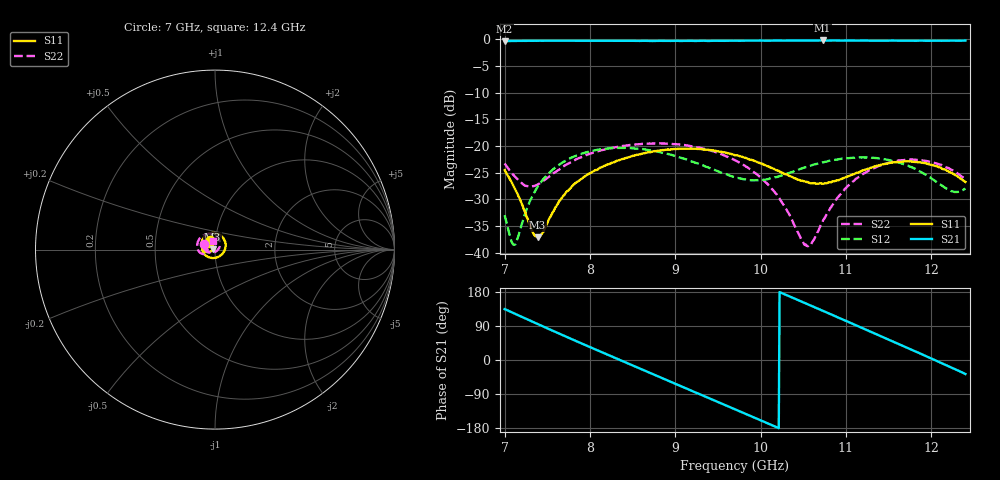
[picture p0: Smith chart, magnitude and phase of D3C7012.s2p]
! 11/4/2020 3:57:07 PM
! C:\USERS\DITOM\DESKTOP\SINGLE JUNCTION ISOLATOR DATA\7.0 - 12.4 GHZ (D3I7012).S2P
! CHANNEL.1
! TR.MEASUREMENT
! CORRECTED.DATA
# GHZ S RI R 50.0
! FREQ.GHZ  S11RE  S11IM  S21RE  S21IM  S12RE  S12IM  S22RE  S22IM
!; PortSelection: Port_12
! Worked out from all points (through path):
!   601 points, 7 GHz to 12.4 GHz, reference 50 ohm
!   highest |S21| = -0.23 dB at 10.73 GHz (marker M1); lowest = -0.4 dB at 7 GHz (marker M2)
!   lowest |S11| = -37.1 dB at 7.387 GHz (marker M3), VSWR 1.03, Z = 48.7 + j0.403 ohm
!   |S11| at or under -10 dB: start of sweep to end of sweep
!   |S22| runs from -38.8 to -19.5 dB; largest |S21 - S12| = 0.98
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7  -0.0303 0.0511  -0.6701 0.6869  0.0224 0.00224  -0.0619 0.0295
7.126  -0.0173 0.0352  -0.5027 0.8218  0.00612 0.0103  -0.0483 0.0174
7.387  -0.0133 0.00413  -0.0823 0.964  0.00224 0.0414  -0.0423 -0.00948
7.639  -0.0279 -0.0123  0.3367 0.908  0.0316 0.0588  -0.0554 -0.0235
7.9  -0.0474 -0.0131  0.6976 0.6714  0.0718 0.0449  -0.0754 -0.022
8.134  -0.063 -0.00263  0.9034 0.3469  0.093 0.00845  -0.0909 -0.00903
8.341  -0.0724 0.0134  0.9661 0.0136  0.0908 -0.0306  -0.0982 0.00975
8.593  -0.0744 0.0389  0.8853 -0.3841  0.0647 -0.0682  -0.0974 0.0365
8.8  -0.0661 0.0613  0.7004 -0.6642  0.0317 -0.0825  -0.088 0.0581
9.034  -0.0458 0.0821  0.3908 -0.8824  -0.00337 -0.0788  -0.068 0.0784
9.277  -0.015 0.0927  0.0122 -0.9655  -0.0273 -0.0623  -0.0392 0.0884
9.7  0.0383 0.0725  -0.6256 -0.7391  -0.0393 -0.0323  0.00978 0.073
10.159  0.0589 0.0158  -0.9674 -0.0918  -0.0467 -0.0196  0.0278 0.0251
10.492  0.0405 -0.0243  -0.8666 0.4415  -0.062 -0.0012  0.0115 -0.00571
10.6  0.0292 -0.0339  -0.7692 0.593  -0.0654 0.00959  0.00214 -0.0122
10.726  0.0146 -0.0419  -0.6261 0.746  -0.0656 0.0251  -0.00991 -0.0167
11.113  -0.0358 -0.0425  -0.0344 0.9696  -0.0338 0.0704  -0.0482 -0.00875
11.5  -0.0683 -0.00873  0.5693 0.7842  0.0307 0.0674  -0.0651 0.0248
11.734  -0.0701 0.015  0.8356 0.4936  0.0559 0.0333  -0.059 0.0454
11.959  -0.0603 0.0311  0.9566 0.1355  0.0516 -0.0081  -0.0442 0.057
12.175  -0.0473 0.0358  0.9408 -0.2298  0.0195 -0.0349  -0.0274 0.057
12.4  -0.0354 0.0295  0.7773 -0.584  -0.0282 -0.0283  -0.0123 0.0467
